FUNCTION "Gest Output" : VOID
TITLE =Gestione Output
AUTHOR : MassimoZ
FAMILY : NovaSrl
VERSION : 0.1

BEGIN
NETWORK
TITLE =R0 = Ripristino Emergenza
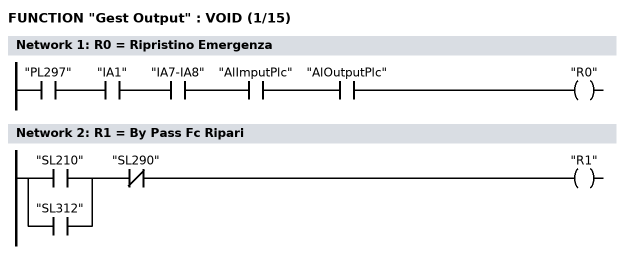
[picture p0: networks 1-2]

      U     "PL297";
      U     "IA1";
      U     "IA7-IA8";
      U     "AlImputPlc";
      U     "AlOutputPlc";
      =     "R0";
NETWORK
TITLE =R1 = By Pass Fc Ripari

      U(    ;
      O     "SL210";
      O     "SL312";
      )     ;
      UN    "SL290";
      =     "R1";
NETWORK
TITLE =R2 = Com Motore Pompa Centralina Idraulica
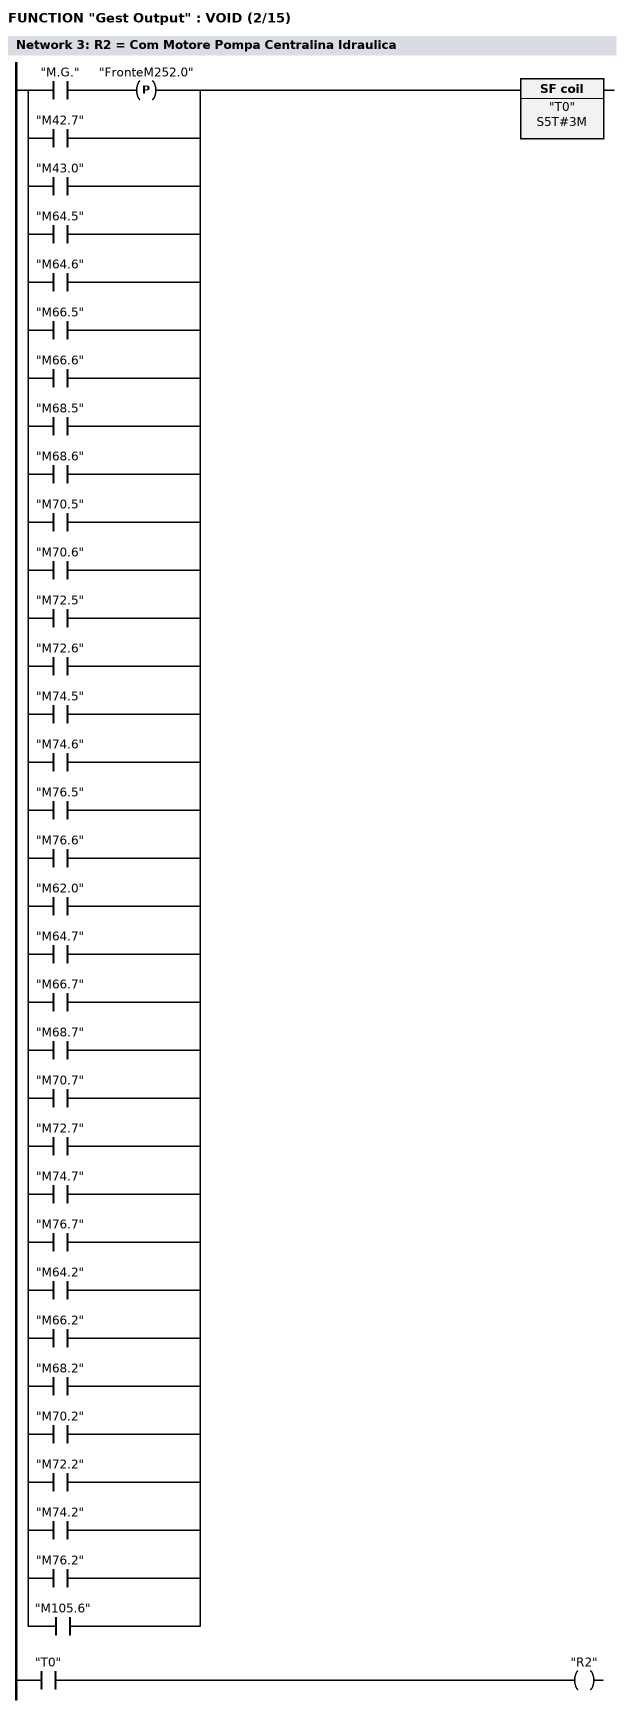
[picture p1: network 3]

      U(    ;
      U     "M.G.";
      FP    "FronteM252.0";
      O     "M42.7";
      O     "M43.0";
      O     "M64.5";
      O     "M64.6";
      O     "M66.5";
      O     "M66.6";
      O     "M68.5";
      O     "M68.6";
      O     "M70.5";
      O     "M70.6";
      O     "M72.5";
      O     "M72.6";
      O     "M74.5";
      O     "M74.6";
      O     "M76.5";
      O     "M76.6";
      O     "M62.0";
      O     "M64.7";
      O     "M66.7";
      O     "M68.7";
      O     "M70.7";
      O     "M72.7";
      O     "M74.7";
      O     "M76.7";
      O     "M64.2";
      O     "M66.2";
      O     "M68.2";
      O     "M70.2";
      O     "M72.2";
      O     "M74.2";
      O     "M76.2";
      O     "M105.6";
      )     ;
      L     S5T#3M;
      SA    "T0";
      NOP   0;
      NOP   0;
      NOP   0;
      U     "T0";
      =     "R2";
NETWORK
TITLE =R3 = Com Motore Nastro Orizzontale
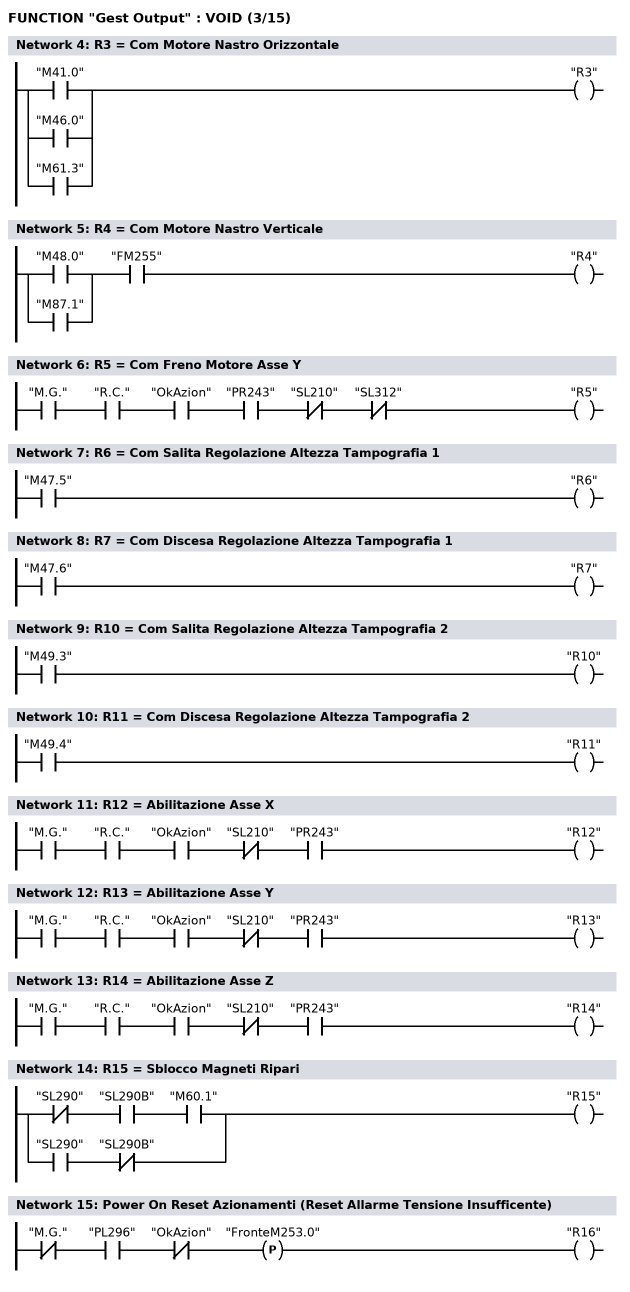
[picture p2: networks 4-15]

      O     "M41.0";
      O     "M46.0";
      O     "M61.3";
      =     "R3";
NETWORK
TITLE =R4 = Com Motore Nastro Verticale

      U(    ;
      O     "M48.0";
      O     "M87.1";
      )     ;
      U     "FM255";
      =     "R4";
NETWORK
TITLE =R5 = Com Freno Motore Asse Y

      U     "M.G.";
      U     "R.C.";
      U     "OkAzion";
      U     "PR243";
      UN    "SL210";
      UN    "SL312";
      =     "R5";
NETWORK
TITLE =R6 = Com Salita Regolazione Altezza Tampografia 1

      U     "M47.5";
      =     "R6";
NETWORK
TITLE =R7 = Com Discesa Regolazione Altezza Tampografia 1

      U     "M47.6";
      =     "R7";
NETWORK
TITLE =R10 = Com Salita Regolazione Altezza Tampografia 2

      U     "M49.3";
      =     "R10";
NETWORK
TITLE =R11 = Com Discesa Regolazione Altezza Tampografia 2

      U     "M49.4";
      =     "R11";
NETWORK
TITLE =R12 = Abilitazione Asse X

      U     "M.G.";
      U     "R.C.";
      U     "OkAzion";
      UN    "SL210";
      U     "PR243";
      =     "R12";
NETWORK
TITLE =R13 = Abilitazione Asse Y

      U     "M.G.";
      U     "R.C.";
      U     "OkAzion";
      UN    "SL210";
      U     "PR243";
      =     "R13";
NETWORK
TITLE =R14 = Abilitazione Asse Z

      U     "M.G.";
      U     "R.C.";
      U     "OkAzion";
      UN    "SL210";
      U     "PR243";
      =     "R14";
NETWORK
TITLE =R15 = Sblocco Magneti Ripari

      UN    "SL290";
      U     "SL290B";
      U     "M60.1";
      O     ;
      U     "SL290";
      UN    "SL290B";
      =     "R15";
NETWORK
TITLE =Power On Reset Azionamenti (Reset Allarme Tensione Insufficente)

      UN    "M.G.";
      U     "PL296";
      UN    "OkAzion";
      FP    "FronteM253.0";
      =     "R16";
NETWORK
TITLE =EV100 = Avanti Cadenziatore in Entrata Zona Foratrice
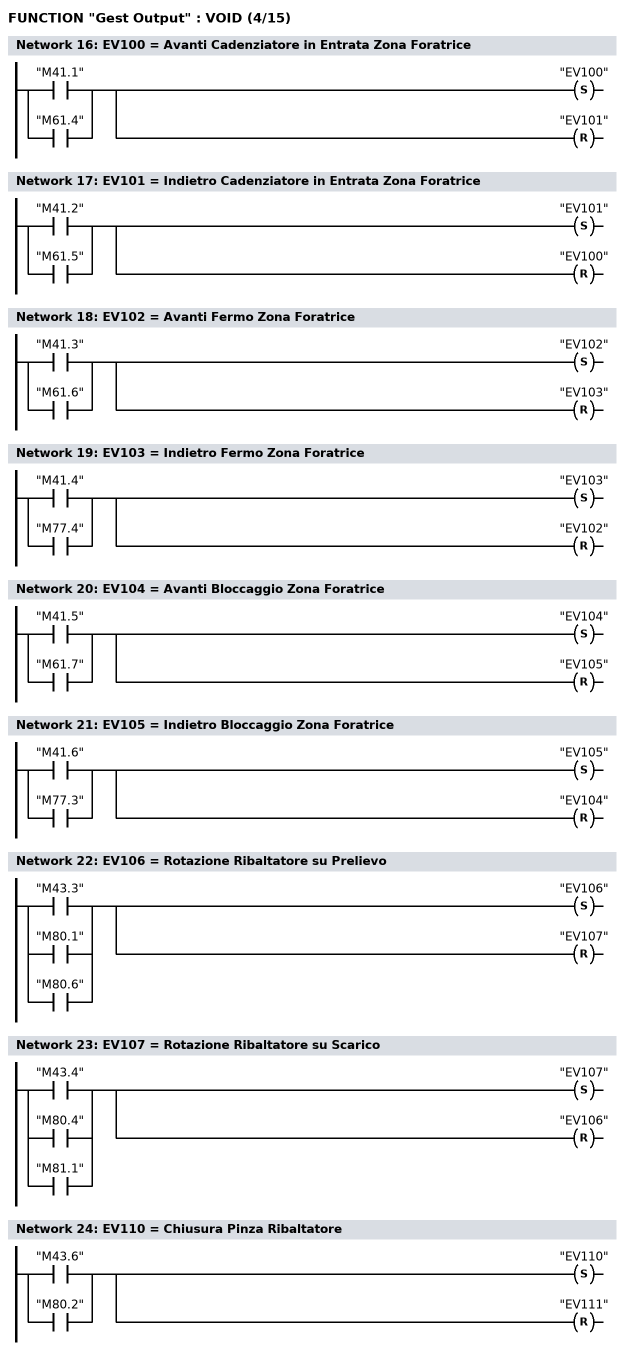
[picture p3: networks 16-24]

      O     "M41.1";
      O     "M61.4";
      S     "EV100";
      R     "EV101";
NETWORK
TITLE =EV101 = Indietro Cadenziatore in Entrata Zona Foratrice

      O     "M41.2";
      O     "M61.5";
      S     "EV101";
      R     "EV100";
NETWORK
TITLE =EV102 = Avanti Fermo Zona Foratrice

      O     "M41.3";
      O     "M61.6";
      S     "EV102";
      R     "EV103";
NETWORK
TITLE =EV103 = Indietro Fermo Zona Foratrice

      O     "M41.4";
      O     "M77.4";
      S     "EV103";
      R     "EV102";
NETWORK
TITLE =EV104 = Avanti Bloccaggio Zona Foratrice

      O     "M41.5";
      O     "M61.7";
      S     "EV104";
      R     "EV105";
NETWORK
TITLE =EV105 = Indietro Bloccaggio Zona Foratrice

      O     "M41.6";
      O     "M77.3";
      S     "EV105";
      R     "EV104";
NETWORK
TITLE =EV106 = Rotazione Ribaltatore su Prelievo

      O     "M43.3";
      O     "M80.1";
      O     "M80.6";
      S     "EV106";
      R     "EV107";
NETWORK
TITLE =EV107 = Rotazione Ribaltatore su Scarico

      O     "M43.4";
      O     "M80.4";
      O     "M81.1";
      S     "EV107";
      R     "EV106";
NETWORK
TITLE =EV110 = Chiusura Pinza Ribaltatore

      O     "M43.6";
      O     "M80.2";
      S     "EV110";
      R     "EV111";
NETWORK
TITLE =EV111 = Apertura Pinza Ribaltatore
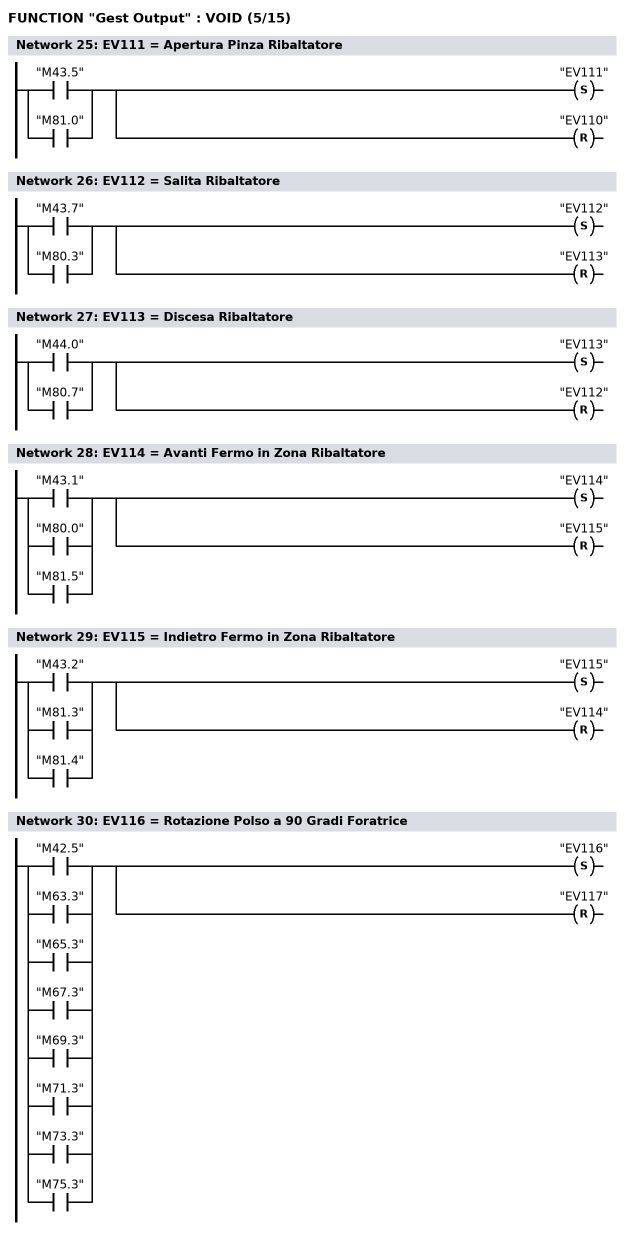
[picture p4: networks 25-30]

      O     "M43.5";
      O     "M81.0";
      S     "EV111";
      R     "EV110";
NETWORK
TITLE =EV112 = Salita Ribaltatore

      O     "M43.7";
      O     "M80.3";
      S     "EV112";
      R     "EV113";
NETWORK
TITLE =EV113 = Discesa Ribaltatore

      O     "M44.0";
      O     "M80.7";
      S     "EV113";
      R     "EV112";
NETWORK
TITLE =EV114 = Avanti Fermo in Zona Ribaltatore

      O     "M43.1";
      O     "M80.0";
      O     "M81.5";
      S     "EV114";
      R     "EV115";
NETWORK
TITLE =EV115 = Indietro Fermo in Zona Ribaltatore

      O     "M43.2";
      O     "M81.3";
      O     "M81.4";
      S     "EV115";
      R     "EV114";
NETWORK
TITLE =EV116 = Rotazione Polso a 90 Gradi Foratrice

      O     "M42.5";
      O     "M63.3";
      O     "M65.3";
      O     "M67.3";
      O     "M69.3";
      O     "M71.3";
      O     "M73.3";
      O     "M75.3";
      S     "EV116";
      R     "EV117";
NETWORK
TITLE =EV117 = Rotazione Polso a 0 Gradi Foratrice
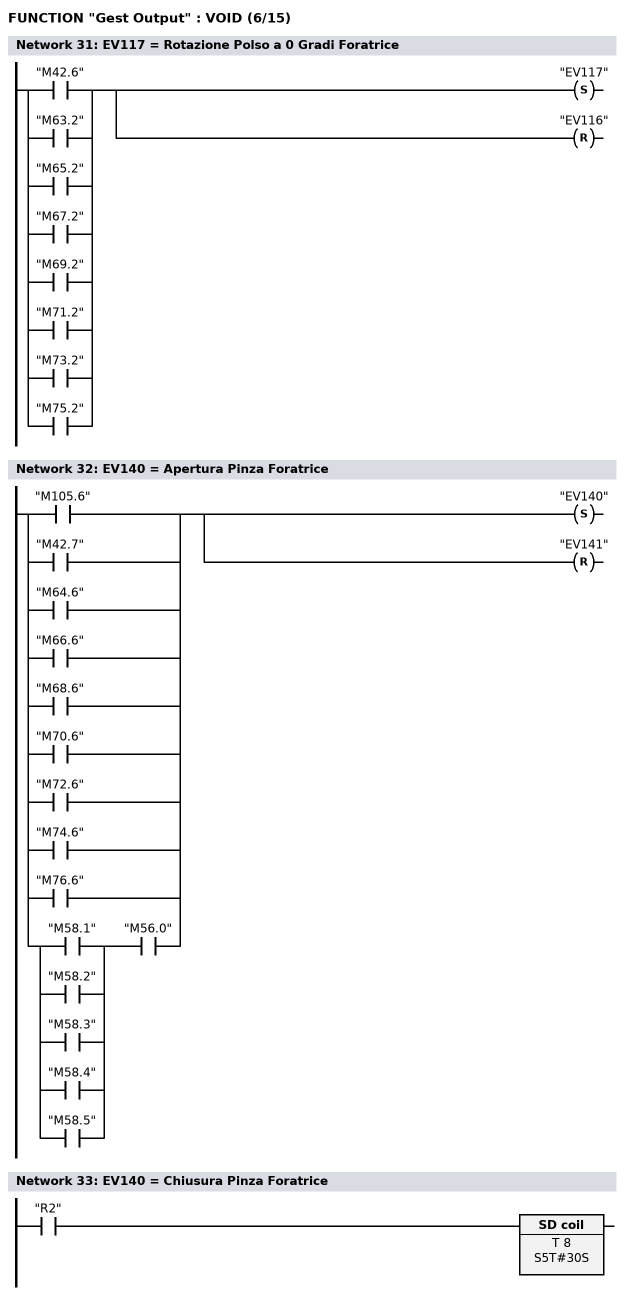
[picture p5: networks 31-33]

      O     "M42.6";
      O     "M63.2";
      O     "M65.2";
      O     "M67.2";
      O     "M69.2";
      O     "M71.2";
      O     "M73.2";
      O     "M75.2";
      S     "EV117";
      R     "EV116";
NETWORK
TITLE =EV140 = Apertura Pinza Foratrice

      O     "M105.6";
      O     "M42.7";
      O     "M64.6";
      O     "M66.6";
      O     "M68.6";
      O     "M70.6";
      O     "M72.6";
      O     "M74.6";
      O     "M76.6";
      O     ;
      U(    ;
      O     "M58.1";
      O     "M58.2";
      O     "M58.3";
      O     "M58.4";
      O     "M58.5";
      )     ;
      U     "M56.0";
      S     "EV140";
      R     "EV141";
NETWORK
TITLE =EV140 = Chiusura Pinza Foratrice

      U     "R2";
      L     S5T#30S;
      SE    T      8;
NETWORK
TITLE =EV160 = Avanti Cadenziatore Entrata Tampografia 1
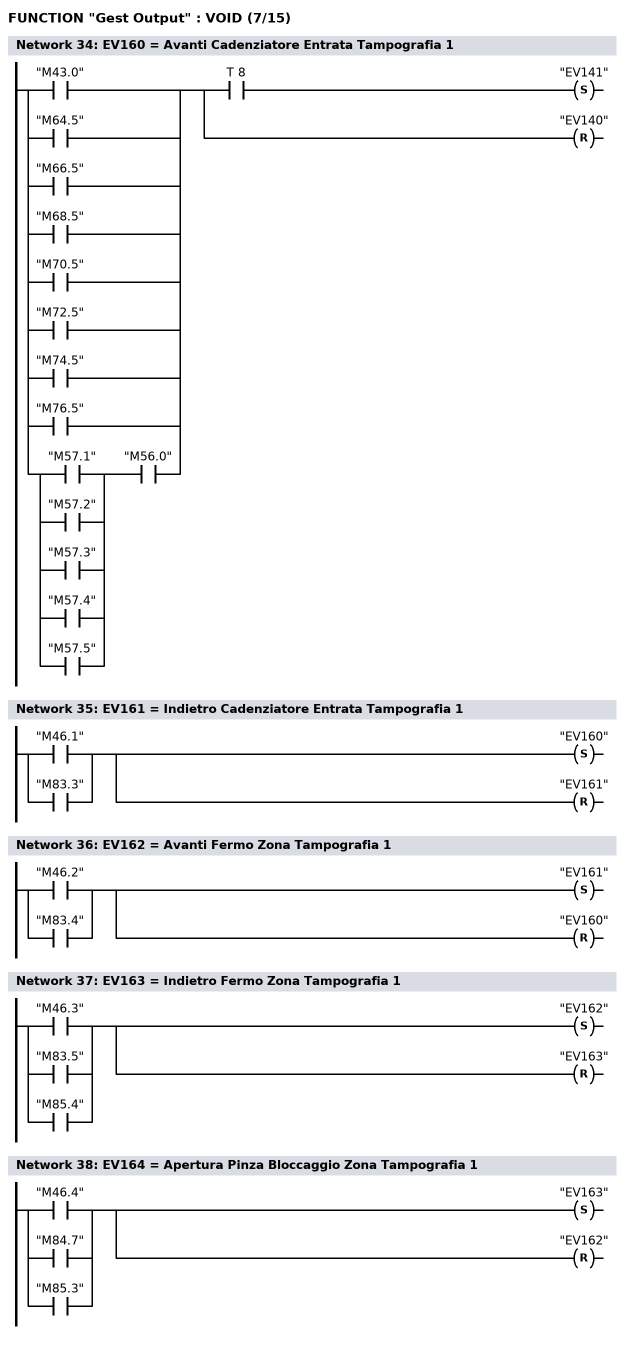
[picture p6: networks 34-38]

      O     "M43.0";
      O     "M64.5";
      O     "M66.5";
      O     "M68.5";
      O     "M70.5";
      O     "M72.5";
      O     "M74.5";
      O     "M76.5";
      O     ;
      U(    ;
      O     "M57.1";
      O     "M57.2";
      O     "M57.3";
      O     "M57.4";
      O     "M57.5";
      )     ;
      U     "M56.0";
      =     L      0.0;
      U     L      0.0;
      U     T      8;
      S     "EV141";
      U     L      0.0;
      BLD   102;
      R     "EV140";
NETWORK
TITLE =EV161 = Indietro Cadenziatore Entrata Tampografia 1

      O     "M46.1";
      O     "M83.3";
      S     "EV160";
      R     "EV161";
NETWORK
TITLE =EV162 = Avanti Fermo Zona Tampografia 1

      O     "M46.2";
      O     "M83.4";
      S     "EV161";
      R     "EV160";
NETWORK
TITLE =EV163 = Indietro Fermo Zona Tampografia 1

      O     "M46.3";
      O     "M83.5";
      O     "M85.4";
      S     "EV162";
      R     "EV163";
NETWORK
TITLE =EV164 = Apertura Pinza Bloccaggio Zona Tampografia 1

      O     "M46.4";
      O     "M84.7";
      O     "M85.3";
      S     "EV163";
      R     "EV162";
NETWORK
TITLE =EV165 = Chiusura Pinza Bloccaggio Zona Tampografia 1
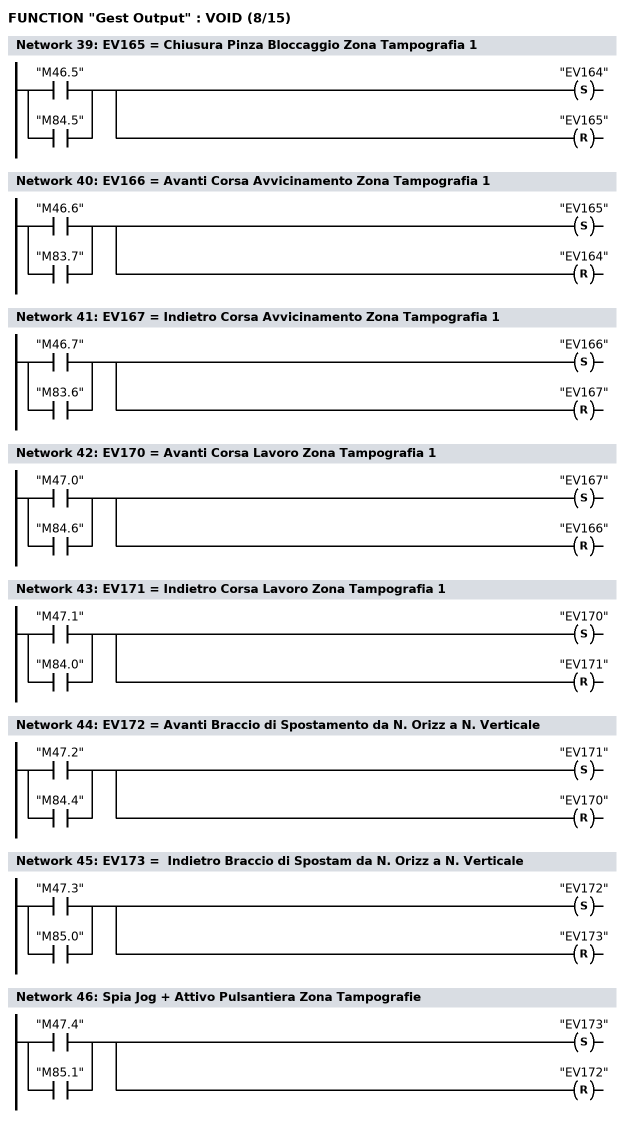
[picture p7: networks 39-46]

      O     "M46.5";
      O     "M84.5";
      S     "EV164";
      R     "EV165";
NETWORK
TITLE =EV166 = Avanti Corsa Avvicinamento Zona Tampografia 1

      O     "M46.6";
      O     "M83.7";
      S     "EV165";
      R     "EV164";
NETWORK
TITLE =EV167 = Indietro Corsa Avvicinamento Zona Tampografia 1

      O     "M46.7";
      O     "M83.6";
      S     "EV166";
      R     "EV167";
NETWORK
TITLE =EV170 = Avanti Corsa Lavoro Zona Tampografia 1

      O     "M47.0";
      O     "M84.6";
      S     "EV167";
      R     "EV166";
NETWORK
TITLE =EV171 = Indietro Corsa Lavoro Zona Tampografia 1

      O     "M47.1";
      O     "M84.0";
      S     "EV170";
      R     "EV171";
NETWORK
TITLE =EV172 = Avanti Braccio di Spostamento da N. Orizz a N. Verticale

      O     "M47.2";
      O     "M84.4";
      S     "EV171";
      R     "EV170";
NETWORK
TITLE =EV173 =  Indietro Braccio di Spostam da N. Orizz a N. Verticale

      O     "M47.3";
      O     "M85.0";
      S     "EV172";
      R     "EV173";
NETWORK
TITLE =Spia Jog + Attivo Pulsantiera Zona Tampografie

      O     "M47.4";
      O     "M85.1";
      S     "EV173";
      R     "EV172";
NETWORK
TITLE =Spia Jog - Attivo Pulsantiera Zona Tampografie
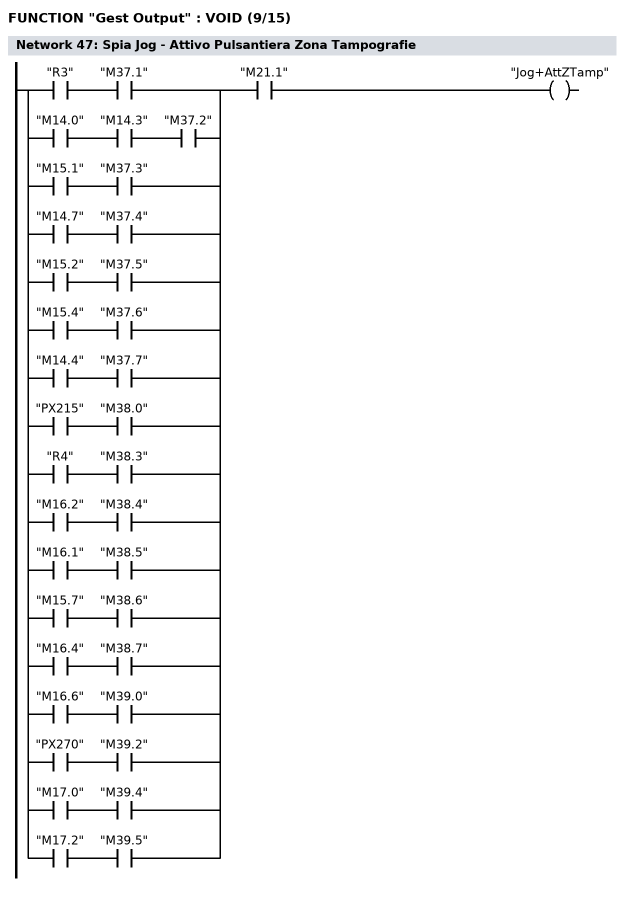
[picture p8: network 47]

      U(    ;
      U     "R3";
      U     "M37.1";
      O     ;
      U     "M14.0";
      U     "M14.3";
      U     "M37.2";
      O     ;
      U     "M15.1";
      U     "M37.3";
      O     ;
      U     "M14.7";
      U     "M37.4";
      O     ;
      U     "M15.2";
      U     "M37.5";
      O     ;
      U     "M15.4";
      U     "M37.6";
      O     ;
      U     "M14.4";
      U     "M37.7";
      O     ;
      U     "PX215";
      U     "M38.0";
      O     ;
      U     "R4";
      U     "M38.3";
      O     ;
      U     "M16.2";
      U     "M38.4";
      O     ;
      U     "M16.1";
      U     "M38.5";
      O     ;
      U     "M15.7";
      U     "M38.6";
      O     ;
      U     "M16.4";
      U     "M38.7";
      O     ;
      U     "M16.6";
      U     "M39.0";
      O     ;
      U     "PX270";
      U     "M39.2";
      O     ;
      U     "M17.0";
      U     "M39.4";
      O     ;
      U     "M17.2";
      U     "M39.5";
      )     ;
      U     "M21.1";
      =     "Jog+AttZTamp";
NETWORK
TITLE =Spia Zona Foratrice a Tampografie in Ciclo
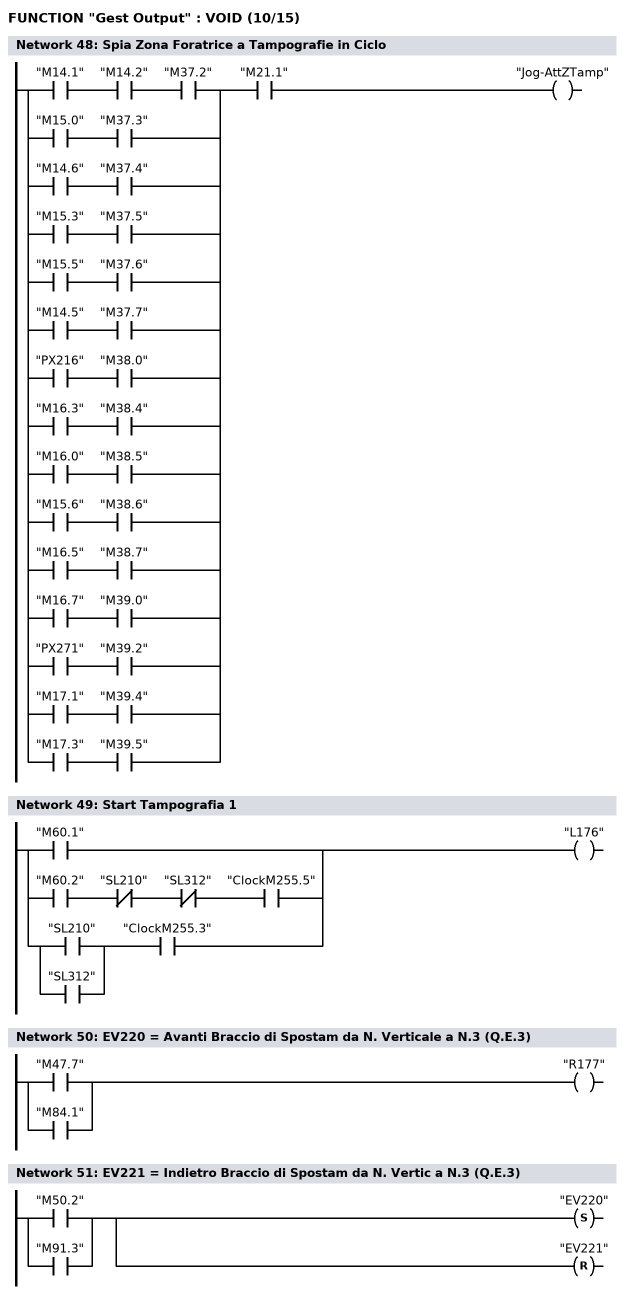
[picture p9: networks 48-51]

      U(    ;
      U     "M14.1";
      U     "M14.2";
      U     "M37.2";
      O     ;
      U     "M15.0";
      U     "M37.3";
      O     ;
      U     "M14.6";
      U     "M37.4";
      O     ;
      U     "M15.3";
      U     "M37.5";
      O     ;
      U     "M15.5";
      U     "M37.6";
      O     ;
      U     "M14.5";
      U     "M37.7";
      O     ;
      U     "PX216";
      U     "M38.0";
      O     ;
      U     "M16.3";
      U     "M38.4";
      O     ;
      U     "M16.0";
      U     "M38.5";
      O     ;
      U     "M15.6";
      U     "M38.6";
      O     ;
      U     "M16.5";
      U     "M38.7";
      O     ;
      U     "M16.7";
      U     "M39.0";
      O     ;
      U     "PX271";
      U     "M39.2";
      O     ;
      U     "M17.1";
      U     "M39.4";
      O     ;
      U     "M17.3";
      U     "M39.5";
      )     ;
      U     "M21.1";
      =     "Jog-AttZTamp";
NETWORK
TITLE =Start Tampografia 1

      O     "M60.1";
      O     ;
      U     "M60.2";
      UN    "SL210";
      UN    "SL312";
      U     "ClockM255.5";
      O     ;
      U(    ;
      O     "SL210";
      O     "SL312";
      )     ;
      U     "ClockM255.3";
      =     "L176";
NETWORK
TITLE =EV220 = Avanti Braccio di Spostam da N. Verticale a N.3 (Q.E.3)

      O     "M47.7";
      O     "M84.1";
      =     "R177";
NETWORK
TITLE =EV221 = Indietro Braccio di Spostam da N. Vertic a N.3 (Q.E.3)

      O     "M50.2";
      O     "M91.3";
      S     "EV220";
      R     "EV221";
NETWORK
TITLE =EV222 = Scorta
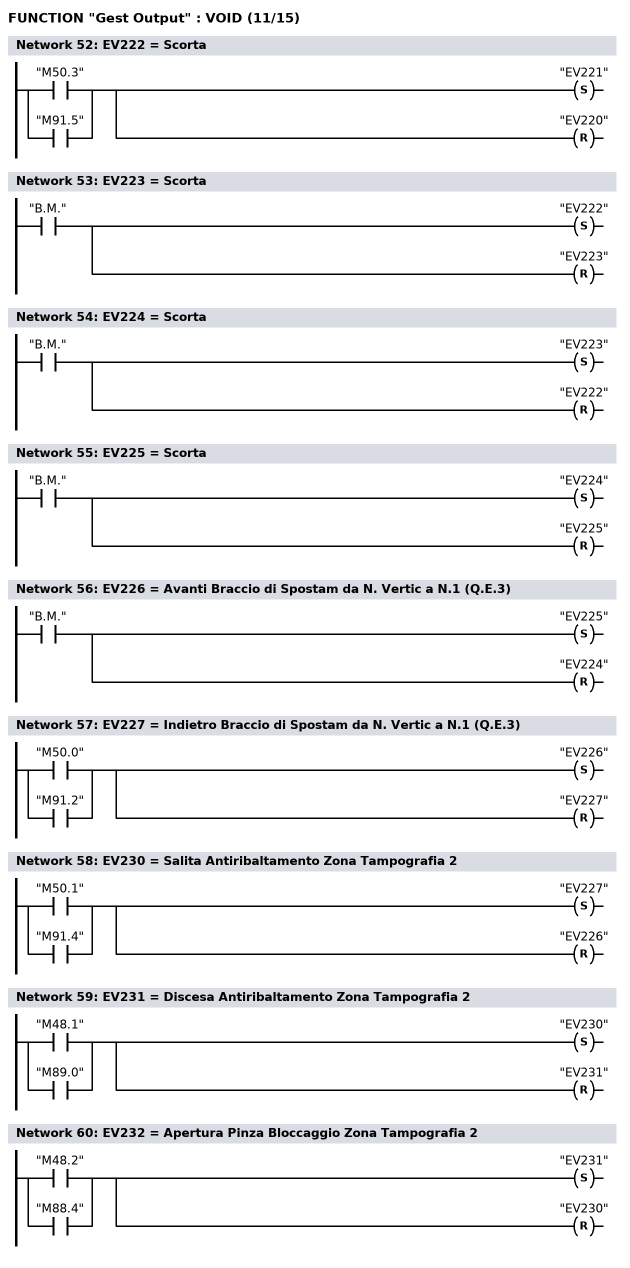
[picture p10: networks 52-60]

      O     "M50.3";
      O     "M91.5";
      S     "EV221";
      R     "EV220";
NETWORK
TITLE =EV223 = Scorta

      U     "B.M.";
      S     "EV222";
      R     "EV223";
NETWORK
TITLE =EV224 = Scorta

      U     "B.M.";
      S     "EV223";
      R     "EV222";
NETWORK
TITLE =EV225 = Scorta

      U     "B.M.";
      S     "EV224";
      R     "EV225";
NETWORK
TITLE =EV226 = Avanti Braccio di Spostam da N. Vertic a N.1 (Q.E.3)

      U     "B.M.";
      S     "EV225";
      R     "EV224";
NETWORK
TITLE =EV227 = Indietro Braccio di Spostam da N. Vertic a N.1 (Q.E.3)

      O     "M50.0";
      O     "M91.2";
      S     "EV226";
      R     "EV227";
NETWORK
TITLE =EV230 = Salita Antiribaltamento Zona Tampografia 2

      O     "M50.1";
      O     "M91.4";
      S     "EV227";
      R     "EV226";
NETWORK
TITLE =EV231 = Discesa Antiribaltamento Zona Tampografia 2

      O     "M48.1";
      O     "M89.0";
      S     "EV230";
      R     "EV231";
NETWORK
TITLE =EV232 = Apertura Pinza Bloccaggio Zona Tampografia 2

      O     "M48.2";
      O     "M88.4";
      S     "EV231";
      R     "EV230";
NETWORK
TITLE =EV233 = Chiusura Pinza Bloccaggio Zona Tampografia 2
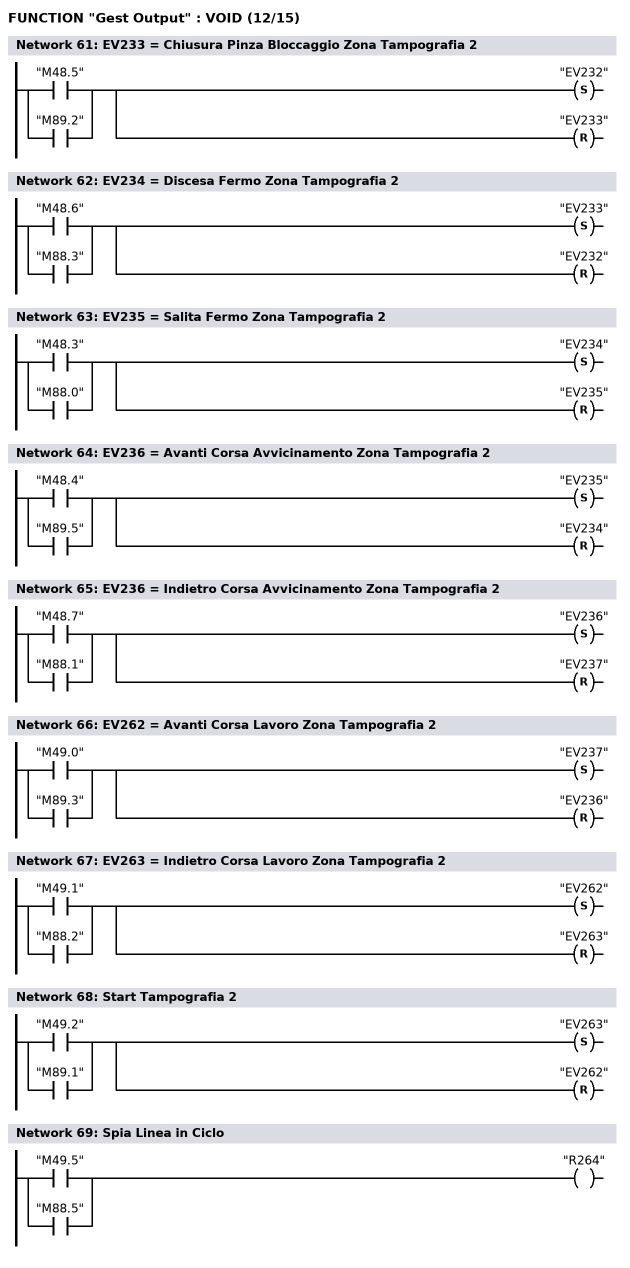
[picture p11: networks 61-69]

      O     "M48.5";
      O     "M89.2";
      S     "EV232";
      R     "EV233";
NETWORK
TITLE =EV234 = Discesa Fermo Zona Tampografia 2

      O     "M48.6";
      O     "M88.3";
      S     "EV233";
      R     "EV232";
NETWORK
TITLE =EV235 = Salita Fermo Zona Tampografia 2

      O     "M48.3";
      O     "M88.0";
      S     "EV234";
      R     "EV235";
NETWORK
TITLE =EV236 = Avanti Corsa Avvicinamento Zona Tampografia 2

      O     "M48.4";
      O     "M89.5";
      S     "EV235";
      R     "EV234";
NETWORK
TITLE =EV236 = Indietro Corsa Avvicinamento Zona Tampografia 2

      O     "M48.7";
      O     "M88.1";
      S     "EV236";
      R     "EV237";
NETWORK
TITLE =EV262 = Avanti Corsa Lavoro Zona Tampografia 2

      O     "M49.0";
      O     "M89.3";
      S     "EV237";
      R     "EV236";
NETWORK
TITLE =EV263 = Indietro Corsa Lavoro Zona Tampografia 2

      O     "M49.1";
      O     "M88.2";
      S     "EV262";
      R     "EV263";
NETWORK
TITLE =Start Tampografia 2

      O     "M49.2";
      O     "M89.1";
      S     "EV263";
      R     "EV262";
NETWORK
TITLE =Spia Linea in Ciclo

      O     "M49.5";
      O     "M88.5";
      =     "R264";
NETWORK
TITLE =Spia Svuotamento
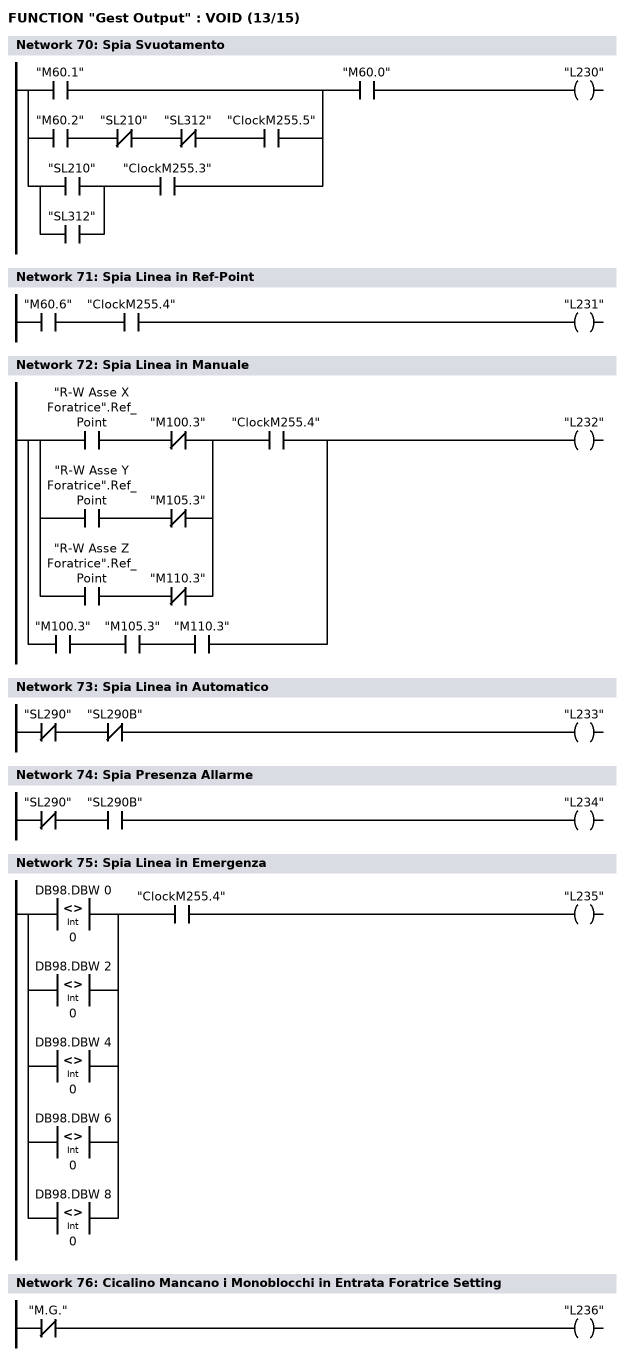
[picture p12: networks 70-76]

      U(    ;
      O     "M60.1";
      O     ;
      U     "M60.2";
      UN    "SL210";
      UN    "SL312";
      U     "ClockM255.5";
      O     ;
      U(    ;
      O     "SL210";
      O     "SL312";
      )     ;
      U     "ClockM255.3";
      )     ;
      U     "M60.0";
      =     "L230";
NETWORK
TITLE =Spia Linea in Ref-Point

      U     "M60.6";
      U     "ClockM255.4";
      =     "L231";
NETWORK
TITLE =Spia Linea in Manuale

      U(    ;
      U     "R-W Asse X Foratrice".Ref_Point;
      UN    "M100.3";
      O     ;
      U     "R-W Asse Y Foratrice".Ref_Point;
      UN    "M105.3";
      O     ;
      U     "R-W Asse Z Foratrice".Ref_Point;
      UN    "M110.3";
      )     ;
      U     "ClockM255.4";
      O     ;
      U     "M100.3";
      U     "M105.3";
      U     "M110.3";
      =     "L232";
NETWORK
TITLE =Spia Linea in Automatico

      UN    "SL290";
      UN    "SL290B";
      =     "L233";
NETWORK
TITLE =Spia Presenza Allarme

      UN    "SL290";
      U     "SL290B";
      =     "L234";
NETWORK
TITLE =Spia Linea in Emergenza

      U(    ;
      O(    ;
      L     DB98.DBW    0;
      L     0;
      <>I   ;
      )     ;
      O(    ;
      L     DB98.DBW    2;
      L     0;
      <>I   ;
      )     ;
      O(    ;
      L     DB98.DBW    4;
      L     0;
      <>I   ;
      )     ;
      O(    ;
      L     DB98.DBW    6;
      L     0;
      <>I   ;
      )     ;
      O(    ;
      L     DB98.DBW    8;
      L     0;
      <>I   ;
      )     ;
      )     ;
      U     "ClockM255.4";
      =     "L235";
NETWORK
TITLE =Cicalino Mancano i Monoblocchi in Entrata Foratrice Setting

      UN    "M.G.";
      =     "L236";
NETWORK
TITLE =Spia Jog + Attivo Zona Foratrice
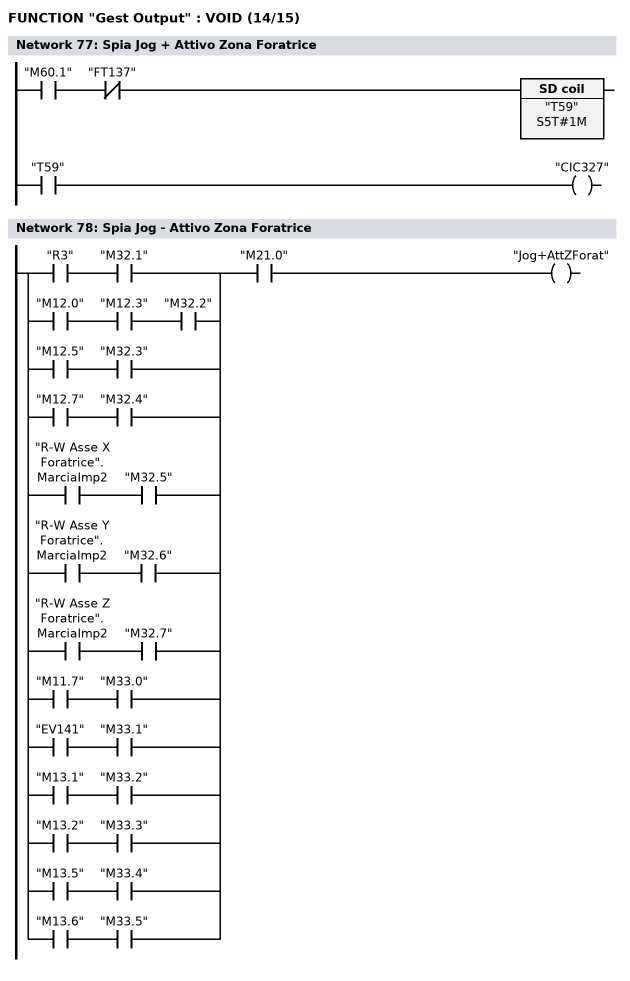
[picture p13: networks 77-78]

      U     "M60.1";
      UN    "FT137";
      L     S5T#1M;
      SE    "T59";
      NOP   0;
      NOP   0;
      NOP   0;
      U     "T59";
      =     "CIC327";
NETWORK
TITLE =Spia Jog - Attivo Zona Foratrice

      U(    ;
      U     "R3";
      U     "M32.1";
      O     ;
      U     "M12.0";
      U     "M12.3";
      U     "M32.2";
      O     ;
      U     "M12.5";
      U     "M32.3";
      O     ;
      U     "M12.7";
      U     "M32.4";
      O     ;
      U     "R-W Asse X Foratrice".MarciaImp2;
      U     "M32.5";
      O     ;
      U     "R-W Asse Y Foratrice".MarciaImp2;
      U     "M32.6";
      O     ;
      U     "R-W Asse Z Foratrice".MarciaImp2;
      U     "M32.7";
      O     ;
      U     "M11.7";
      U     "M33.0";
      O     ;
      U     "EV141";
      U     "M33.1";
      O     ;
      U     "M13.1";
      U     "M33.2";
      O     ;
      U     "M13.2";
      U     "M33.3";
      O     ;
      U     "M13.5";
      U     "M33.4";
      O     ;
      U     "M13.6";
      U     "M33.5";
      )     ;
      U     "M21.0";
      =     "Jog+AttZForat";
NETWORK
TITLE =Caricamento Stato Output nella DB100
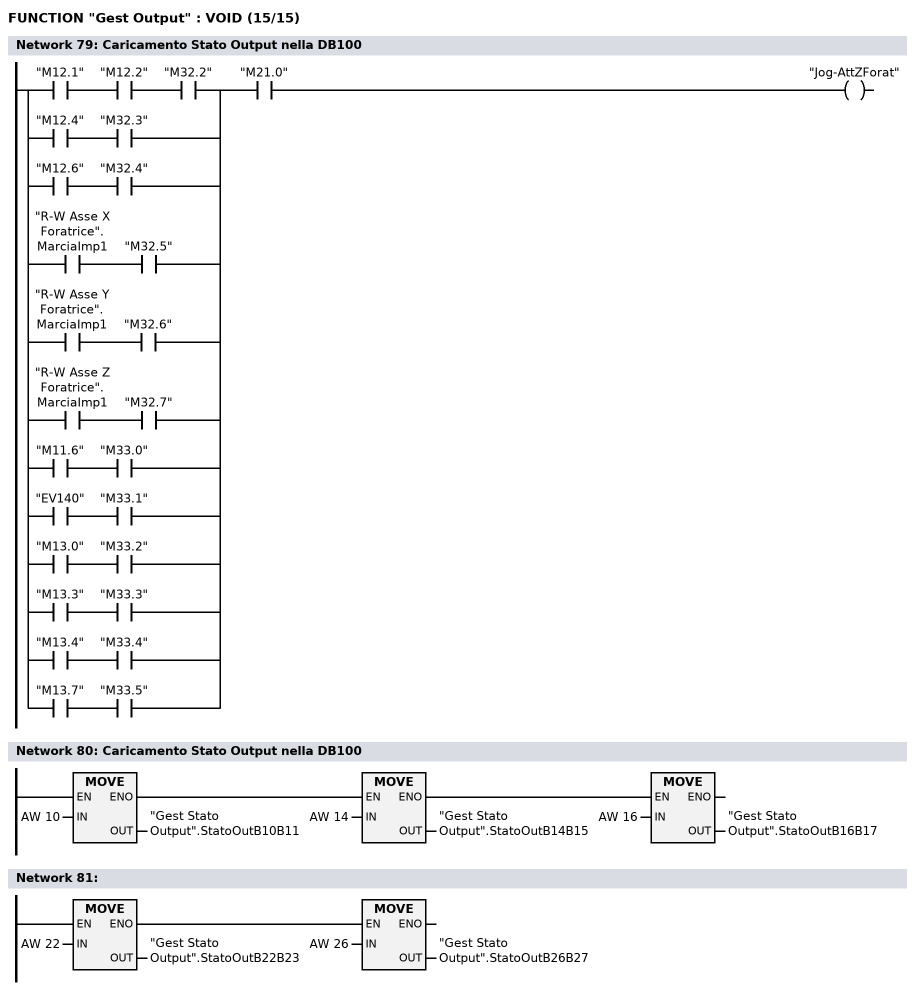
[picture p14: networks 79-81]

      U(    ;
      U     "M12.1";
      U     "M12.2";
      U     "M32.2";
      O     ;
      U     "M12.4";
      U     "M32.3";
      O     ;
      U     "M12.6";
      U     "M32.4";
      O     ;
      U     "R-W Asse X Foratrice".MarciaImp1;
      U     "M32.5";
      O     ;
      U     "R-W Asse Y Foratrice".MarciaImp1;
      U     "M32.6";
      O     ;
      U     "R-W Asse Z Foratrice".MarciaImp1;
      U     "M32.7";
      O     ;
      U     "M11.6";
      U     "M33.0";
      O     ;
      U     "EV140";
      U     "M33.1";
      O     ;
      U     "M13.0";
      U     "M33.2";
      O     ;
      U     "M13.3";
      U     "M33.3";
      O     ;
      U     "M13.4";
      U     "M33.4";
      O     ;
      U     "M13.7";
      U     "M33.5";
      )     ;
      U     "M21.0";
      =     "Jog-AttZForat";
NETWORK
TITLE =Caricamento Stato Output nella DB100

      U(    ;
      U(    ;
      L     AW    10;
      T     "Gest Stato Output".StatoOutB10B11;
      SET   ;
      SAVE  ;
      CLR   ;
      U     BIE;
      )     ;
      SPBNB _001;
      L     AW    14;
      T     "Gest Stato Output".StatoOutB14B15;
      SET   ;
      SAVE  ;
      CLR   ;
_001: U     BIE;
      )     ;
      SPBNB _002;
      L     AW    16;
      T     "Gest Stato Output".StatoOutB16B17;
_002: NOP   0;
NETWORK
TITLE =

      U(    ;
      L     AW    22;
      T     "Gest Stato Output".StatoOutB22B23;
      SET   ;
      SAVE  ;
      CLR   ;
      U     BIE;
      )     ;
      SPBNB _003;
      L     AW    26;
      T     "Gest Stato Output".StatoOutB26B27;
_003: NOP   0;
END_FUNCTION

